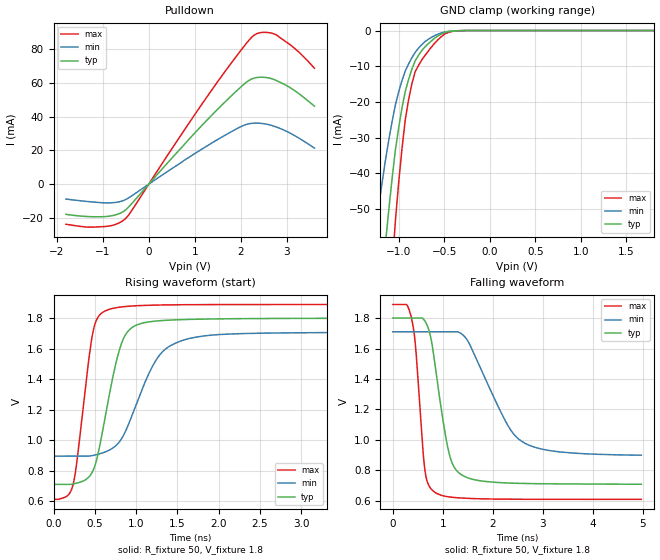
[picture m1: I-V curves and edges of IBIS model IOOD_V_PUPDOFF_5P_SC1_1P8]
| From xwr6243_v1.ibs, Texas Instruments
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|ODF_ADDON_ULPRX; CSI2_TXM[1], CSI2_TXP[1], CSI2_TXP[2], CSI2_TXM[2], CSI2_TXM[3], CSI2_TXP[3]],
|ULTRA LOWER POWER  Receiver
|   Model Cell IOOD_V_PUPDOFF_5P_SC1_1P8
|IOOD_V_PUPDOFF_5P_SC1_1P8
[Model]   IOOD_V_PUPDOFF_5P_SC1_1P8
Model_type   I/O_open_drain
Polarity   Non-Inverting
Enable   Active-Low
Vinl =  0.63
Vinh =  1.17
Cref =  15pF
Rref =  100.0000M
Vref =  0V
Vmeas =  0.9
|   typ   min   max
C_comp   2.233931p   2.204415p   2.290246p
[Model Spec]
Vinl   0.63   0.5985   0.6615
Vinh   1.17   1.1115   1.2285
[Temperature Range]   25   125   -40
[Voltage Range]   1.8   1.71   1.89
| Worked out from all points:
|   slope of the pulldown table from 0 to 0.27 V, typ, clamps not added: 32.2 ohm
|   GND clamp passes 1 mA (typ) near -0.53 V on its own axis
|   rising waveform, R_fixture 50, V_fixture 1.8: 20-80 % time 246ps typ, 396ps min, 169ps max; typ from 0.709 V to 1.8 V
|   falling waveform, R_fixture 50, V_fixture 1.8: 20-80 % time 308ps typ, 718ps min, 171ps max; typ from 1.8 V to 0.709 V
| Where Nom  PVT is Nominal Process, 1.8V, 25C
|   Fast PVT is Strong Process,  1.89V, -40C
|   Slow PVT is Weak Process,   1.71V, 125C
[Pulldown]
|   voltage   I(typ)   I(min)   I(max)
-1.8V     -17.92mA   -8.85mA    -23.8mA
-1.309V   -19.26mA   -10.37mA   -25.5mA
-927.3mV  -19.22mA   -11.12mA   -25.08mA
-654.5mV  -17.65mA   -10.56mA   -23.13mA
-490.9mV  -14.97mA   -8.985mA   -20.05mA
1.364V    40.78mA    24.32mA    55.7mA
2.073V    59.41mA    35mA       81.91mA
2.291V    62.96mA    36.2mA     88.48mA
2.509V    63.41mA    35.84mA    90.12mA
2.782V    61.38mA    33.82mA    88.42mA
3.218V    54.59mA    28.02mA    79.45mA
3.6V      46.26mA    21.39mA    68.79mA
[GND_clamp]
|   voltage   I(typ)   I(min)   I(max)
-1.8V     -270.2mA   -170.2mA   -430.1mA
-1.255V   -91.66mA   -55.91mA   -148.4mA
-1.145V   -59.91mA   -36.45mA   -97.09mA
-1.109V   -50.48mA   -30.83mA   -81.55mA
-1.073V   -41.73mA   -25.65mA   -67.05mA
-1.036V   -33.66mA   -20.92mA   -53.59mA
-927.3mV  -17.07mA   -11.35mA   -25.04mA
-854.5mV  -10.86mA   -7.617mA   -14.91mA
-781.8mV  -6.919mA   -4.945mA   -9.771mA
-636.4mV  -2.823mA   -1.868mA   -4.529mA
-381.8mV  -84.73uA   -78.82uA   -126.1uA
1.8V      19.3nA     350.9nA    215.8nA
[Ramp]
| variable   typ   min   max
dV/dt_f 0.66170167/0.31099078n 0.49657778/0.73394202n 0.77361898/0.17271731n
dV/dt_r 0.65944933/0.43266271n 0.50305793/0.9625316n 0.77800654/0.24641056n
R_load = 50
[Rising Waveform]
R_fixture = 50
V_fixture = 1.8
V_fixture_min = 1.71
V_fixture_max = 1.89
|   time   V(typ)   V(min)   V(max)
0s        709.3mV    894.5mV    611.4mV
234.6ps   711.5mV    894.5mV    703.8mV
472.5ps   793.4mV    898.9mV    1.696V
530.6ps   889.7mV    906mV      1.8V
629.4ps   1.164V     923.1mV    1.849V
776.9ps   1.552V     975.4mV    1.871V
893ps     1.709V     1.085V     1.878V
1.246ns   1.782V     1.529V     1.886V
1.554ns   1.791V     1.653V     1.888V
4.974ns   1.8V       1.708V     1.89V
[Falling Waveform]
R_fixture = 50
V_fixture = 1.8
V_fixture_min = 1.71
V_fixture_max = 1.89
|   time   V(typ)   V(min)   V(max)
0s        1.8V       1.71V      1.889V
275ps     1.8V       1.71V      1.889V
378.3ps   1.8V       1.71V      1.793V
458.3ps   1.8V       1.71V      1.601V
639.6ps   1.782V     1.71V      808.7mV
817.6ps   1.558V     1.71V      661.9mV
1.117ns   924.6mV    1.71V      626.1mV
1.374ns   771.3mV    1.697V     618.4mV
2.562ns   714.5mV    994.7mV    610.4mV
4.974ns   709mV      899.8mV    610mV
